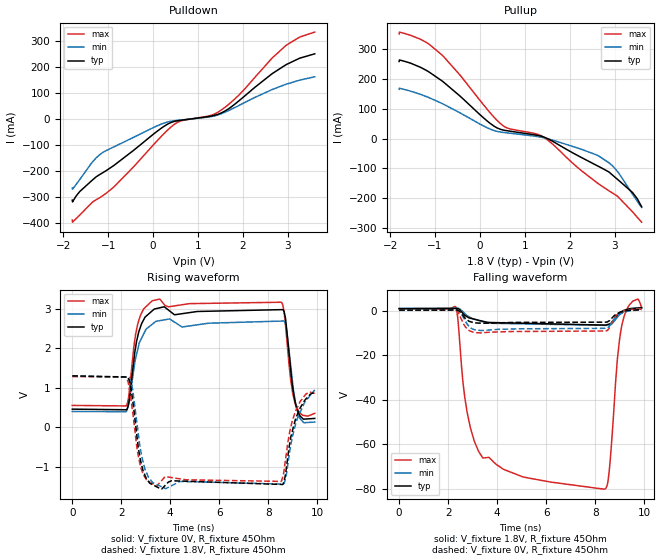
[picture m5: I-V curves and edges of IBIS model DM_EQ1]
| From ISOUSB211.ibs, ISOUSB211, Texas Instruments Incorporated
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[Model]   DM_EQ1
Model_type   Output
Polarity   Inverting
Vmeas = 0.2
Vref = 0
Cref = 15pF
Rref = 45
|   typ   min   max
C_comp   5pF   3pF   8pF
[Voltage Range]   1.8   1.71   1.89
[Temperature Range]   27   150   -40
[Pullup Reference]   1.8   1.71   1.89
[Pulldown Reference]   0   0   0
[Power Clamp Reference]   1.8   1.71   1.89
[GND Clamp Reference]   0   0   0
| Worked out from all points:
|   slope of the pulldown table from 0 to 0.27 V, typ, clamps not added: 7.95 ohm
|   slope of the pullup table from 0 to 0.27 V, typ, clamps not added: 7.94 ohm
|   falling waveform, V_fixture 1.8V, R_fixture 45Ohm: 20-80 % time 296ps typ, 197ps min, 52.8ps max; typ from 0.895 V to 1.3 V
|   rising waveform, V_fixture 0V, R_fixture 45Ohm: 20-80 % time 112ps typ, 126ps min, 92.4ps max; typ from 0.46 V to 0.225 V
|   rising waveform, V_fixture 1.8V, R_fixture 45Ohm: 20-80 % time 97.9ps typ, 103ps min, 94.6ps max; typ from 1.3 V to 0.895 V
|   falling waveform, V_fixture 0V, R_fixture 45Ohm: 20-80 % time 223ps typ, 148ps min, 108ps max; typ from 0.225 V to 0.46 V
[Pulldown]
|   Voltage   I(typ)   I(min)   I(max)
-1.8V     -312.3mA   -266.2mA   -388.8mA
-1.795V   -319mA     -269.8mA   -396.8mA
-1.633V   -278.9mA   -232.8mA   -369.2mA
-1.179V   -212.7mA   -136mA     -301.6mA
-865.8mV  -177.8mA   -106.8mA   -260mA
73.8mV    -49.63mA   -27.98mA   -87.09mA
538.2mV   -7.266mA   -5.626mA   -13.71mA
1.294V    10.85mA    9.019mA    13.98mA
1.521V    23.18mA    20.15mA    34.45mA
1.899V    67.71mA    50.57mA    89.7mA
2.947V    206.8mA    132.3mA    280.4mA
3.6V      250.2mA    161.9mA    333.6mA
[Pullup]
|   Voltage   I(typ)   I(min)   I(max)
-1.8V     259.8mA    166.3mA    352.1mA
-1.795V   264.8mA    169.7mA    358.5mA
-1.325V   240.1mA    149.1mA    334.3mA
-849.6mV  194.9mA    118.9mA    282mA
381.6mV   36.3mA     24.84mA    61.51mA
613.8mV   26.64mA    19.55mA    35.63mA
1.402V    6.733mA    3.773mA    6.537mA
2.612V    -90.76mA   -55.24mA   -148.5mA
2.876V    -112.3mA   -81.28mA   -175.5mA
3.065V    -136.9mA   -110.7mA   -193.6mA
3.4V      -181.3mA   -187.3mA   -246.2mA
3.6V      -228.6mA   -231.2mA   -280.5mA
[Ramp]
R_load = 45
|   typ   min   max
dV/dt_r   0.140808/1.17096e-09   0.160407/1.16936e-10   0.120509/1.00252e-10
dV/dt_f   0.243789/7.35529e-09   0.210518/7.51005e-09   0.256824/1.59773e-09
[Falling Waveform]
V_fixture = 1.8V
V_fixture_min = 1.71V
V_fixture_max = 1.89V
R_fixture = 45Ohm
C_fixture = 0F
|   Time   V(typ)   V(min)   V(max)
0s        895mV      947.6mV    856.5mV
2.312ns   992.2mV    1.058V     1.665V
2.771ns   -2.717V    -2.244V    -45.33V
3.414ns   -4.776V    -4.959V    -66.1V
8.363ns   -6.485V    -6.609V    -80.17V
8.563ns   -6.077V    -6.326V    -73.52V
8.902ns   -2.154V    -3.086V    -22.82V
9.102ns   -323.3mV   -953.7mV   -6.152V
9.535ns   1V         909mV      4.207V
9.9ns     1.301V     1.298V     1.285V
[Rising Waveform]
V_fixture = 0V
V_fixture_min = 0V
V_fixture_max = 0V
R_fixture = 45Ohm
C_fixture = 0F
|   Time   V(typ)   V(min)   V(max)
0s        459.5mV    400.3mV    553.4mV
2.207ns   443.8mV    395mV      540.8mV
2.663ns   2.277V     1.945V     2.587V
3.258ns   2.942V     2.603V     3.196V
8.523ns   2.975V     2.686V     3.163V
8.755ns   2.458V     2.451V     2.242V
8.924ns   1.422V     1.528V     1.174V
9.102ns   641.2mV    662.8mV    589.5mV
9.451ns   206.5mV    116mV      299.1mV
9.9ns     224.9mV    133mV      352.5mV
[Rising Waveform]
V_fixture = 1.8V
V_fixture_min = 1.71V
V_fixture_max = 1.89V
R_fixture = 45Ohm
C_fixture = 0F
|   Time   V(typ)   V(min)   V(max)
0s        1.301V     1.298V     1.285V
2.268ns   1.272V     1.266V     1.167V
2.462ns   701mV      959.6mV    409.7mV
2.806ns   -887mV     -627.1mV   -1.032V
3.111ns   -1.368V    -1.261V    -1.362V
3.63ns    -1.564V    -1.499V    -1.359V
8.619ns   -1.42V     -1.436V    -1.185V
8.881ns   -399.1mV   -600.6mV   -97.37mV
9.11ns    198.9mV    57.17mV    403.2mV
9.9ns     895mV      947.6mV    856.5mV
[Falling Waveform]
|Gnd
V_fixture = 0V
V_fixture_min = 0V
V_fixture_max = 0V
R_fixture = 45Ohm
C_fixture = 0F
|   Time   V(typ)   V(min)   V(max)
0s        224.9mV    133mV      352.5mV
2.307ns   269.6mV    193.8mV    404.4mV
2.503ns   -816.2mV   -685.1mV   -2.938V
2.784ns   -4.269V    -6.112V    -8.317V
2.985ns   -5.225V    -8.186V    -9.56V
3.319ns   -5.638V    -8.893V    -9.996V
8.436ns   -5.175V    -7.954V    -9.14V
8.817ns   -1.935V    -3.394V    -2.788V
8.998ns   -799.1mV   -1.672V    -967mV
9.9ns     459.5mV    400.3mV    553.4mV
